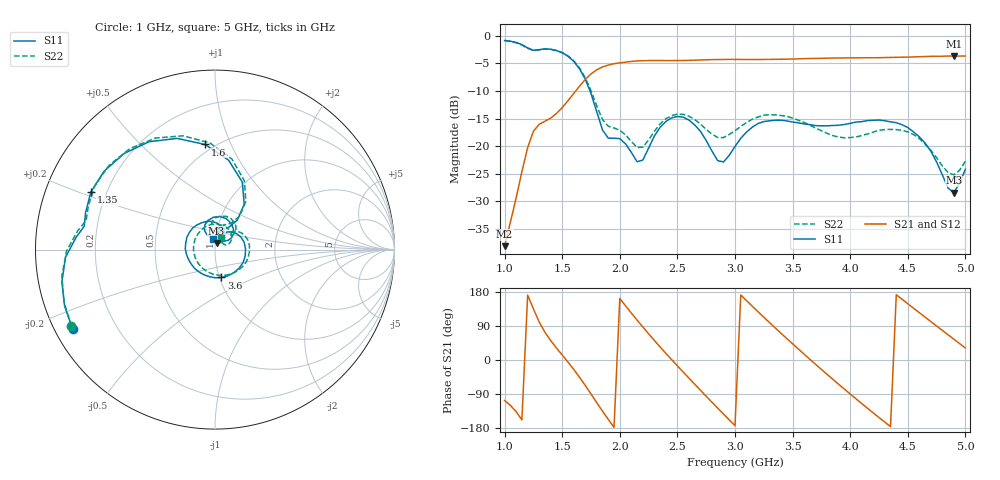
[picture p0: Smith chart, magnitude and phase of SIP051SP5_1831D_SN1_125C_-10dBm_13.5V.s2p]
# GHz  S  dB  R  50
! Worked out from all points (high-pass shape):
!   81 points, 1 GHz to 5 GHz, reference 50 ohm
!   highest |S21| = -3.65 dB at 4.9 GHz (marker M1); lowest = -38.1 dB at 1 GHz (marker M2)
!   |S21| within 3 dB of the highest: 1.767 GHz to end of sweep
!   lowest |S11| = -28.4 dB at 4.9 GHz (marker M3), VSWR 1.08, Z = 50.7 + j3.76 ohm
!   |S11| at or under -10 dB: 1.742 GHz to end of sweep
!   |S22| runs from -25.2 to -0.9 dB; largest |S21 - S12| = 0.0021
!   S11 on the Smith chart (normalised r, x): 1 GHz: 0.05, -0.26; 1.35 GHz: 0.14, +0.22; 1.6 GHz: 0.45, +0.80; 3.6 GHz: 1.02, -0.33; 5 GHz: 0.97, +0.12
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1  -0.83 -150.7  -38.10 -106.8  -38.22 -105.6  -0.86 -152.0
1.2  -2.19 175.0  -20.25 171.4  -20.26 171.5  -2.24 172.3
1.35  -2.36 155.1  -15.47 73.2  -15.47 73.1  -2.40 152.1
1.6  -4.61 95.4  -10.44 -24.8  -10.42 -24.8  -4.52 92.7
1.7  -7.83 68.0  -7.90 -67.2  -7.90 -67.2  -7.59 66.9
1.85  -17.06 59.1  -5.62 -135.0  -5.62 -135.1  -15.16 58.2
2  -18.62 79.3  -4.88 162.5  -4.86 162.4  -17.10 70.8
2.15  -22.80 90.9  -4.54 105.3  -4.55 105.4  -20.21 79.0
2.35  -16.56 112.5  -4.47 34.4  -4.45 34.5  -15.94 95.3
2.5  -14.59 81.4  -4.47 -15.5  -4.46 -15.5  -14.19 71.7
2.7  -17.29 40.7  -4.36 -79.7  -4.35 -79.7  -15.97 43.0
2.85  -22.60 41.0  -4.29 -127.0  -4.28 -127.0  -18.42 42.0
3  -20.04 60.5  -4.27 -173.2  -4.26 -173.3  -17.18 46.5
3.15  -16.54 37.1  -4.28 141.9  -4.28 141.9  -15.09 31.2
3.3  -15.39 1.3  -4.26 98.6  -4.26 98.6  -14.28 6.9
3.6  -15.95 -77.2  -4.13 15.4  -4.13 15.4  -15.68 -54.3
3.7  -16.26 -102.5  -4.09 -11.5  -4.08 -11.5  -16.71 -79.8
4  -15.85 -171.3  -3.99 -89.7  -4.00 -89.7  -18.42 -174.3
4.35  -15.57 115.5  -3.91 -175.9  -3.92 -175.8  -16.95 86.6
4.65  -19.41 58.7  -3.75 113.2  -3.75 113.2  -19.59 30.2
4.9  -28.41 77.0  -3.65 54.8  -3.66 54.8  -25.17 43.4
5  -24.15 102.6  -3.65 31.7  -3.66 31.7  -22.72 60.6
